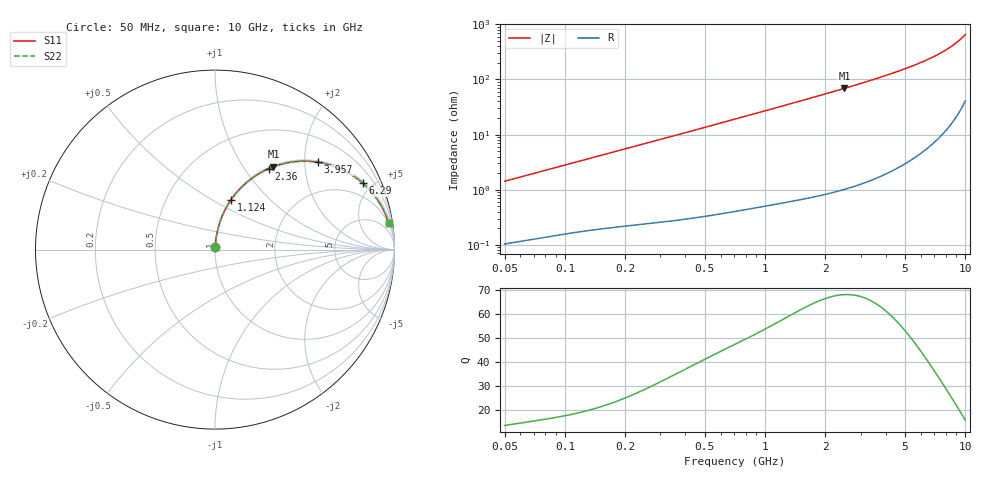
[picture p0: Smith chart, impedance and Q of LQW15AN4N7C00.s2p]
!Murata Part Number: LQW15AN4N7C00
!These Parameters are Measured in Series Mode Connection
!  o--[Z]--o
!Port1  Port2
!  o-------o
!Freq. Start=50[MHz] Stop=10[GHz], 401[Steps]
# Hz S RI R 50
!Freq.(Hz)	S 11(Real)	S 11(Imag)	S 21(Real)	S 21(Imag)	S 12(Real)	S 12(Imag)	S 22(Real)	S 22(Imag)
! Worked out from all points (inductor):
!   401 points, 50 MHz to 10 GHz, reference 50 ohm
!   read as one part in series: L = 4.5 nH near 51.34 MHz
!   highest Q = 67.9 at 2.489 GHz (marker M1), where L = 4.42 nH
!   S11 on the Smith chart (normalised r, x): 50 MHz: 1.00, +0.03; 1.124 GHz: 1.01, +0.61; 2.36 GHz: 1.02, +1.31; 3.957 GHz: 1.04, +2.33; 6.29 GHz: 1.10, +4.39; 10 GHz: 2, +13
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5e7  0.00124 0.0142  0.9988 -0.0142  0.9988 -0.0142  0.00124 0.0142
1.214486e8  0.00288 0.0335  0.9971 -0.0335  0.9971 -0.0335  0.00288 0.0335
2.949953e8  0.00891 0.0794  0.9911 -0.0794  0.9911 -0.0794  0.00891 0.0794
4.689809e8  0.0189 0.1244  0.9811 -0.1244  0.9811 -0.1244  0.0189 0.1244
7.071068e8  0.0389 0.1831  0.9611 -0.1831  0.9611 -0.1831  0.0389 0.1831
9.094607e8  0.061 0.2298  0.939 -0.2298  0.939 -0.2298  0.061 0.2298
1.124152e9  0.0888 0.2757  0.9112 -0.2757  0.9112 -0.2757  0.0888 0.2757
1.408053e9  0.1314 0.3297  0.8686 -0.3297  0.8686 -0.3297  0.1314 0.3297
1.717543e9  0.1835 0.3794  0.8165 -0.3794  0.8165 -0.3794  0.1835 0.3794
2.013439e9  0.2369 0.4177  0.7631 -0.4177  0.7631 -0.4177  0.2369 0.4177
2.360312e9  0.3014 0.4516  0.6986 -0.4516  0.6986 -0.4516  0.3014 0.4516
2.488741e9  0.3254 0.4612  0.6746 -0.4612  0.6746 -0.4612  0.3254 0.4612
3.158828e9  0.4467 0.4897  0.5533 -0.4897  0.5533 -0.4897  0.4467 0.4897
3.956578e9  0.5745 0.4864  0.4255 -0.4864  0.4255 -0.4864  0.5745 0.4864
4.171863e9  0.6051 0.4805  0.3949 -0.4805  0.3949 -0.4805  0.6051 0.4805
5.088839e9  0.7167 0.4411  0.2833 -0.4411  0.2833 -0.4411  0.7167 0.4411
6.290134e9  0.8222 0.3706  0.1778 -0.3706  0.1778 -0.3706  0.8222 0.3706
7.181012e9  0.8771 0.3143  0.1229 -0.3143  0.1229 -0.3143  0.8771 0.3143
8.090191e9  0.9179 0.2573  0.0821 -0.2573  0.0821 -0.2573  0.9179 0.2573
8.876195e9  0.9436 0.2099  0.0564 -0.2099  0.0564 -0.2099  0.9436 0.2099
9.738562e9  0.9637 0.1605  0.0363 -0.1605  0.0363 -0.1605  0.9637 0.1605
1e10  0.9685 0.1461  0.0315 -0.1461  0.0315 -0.1461  0.9685 0.1461
